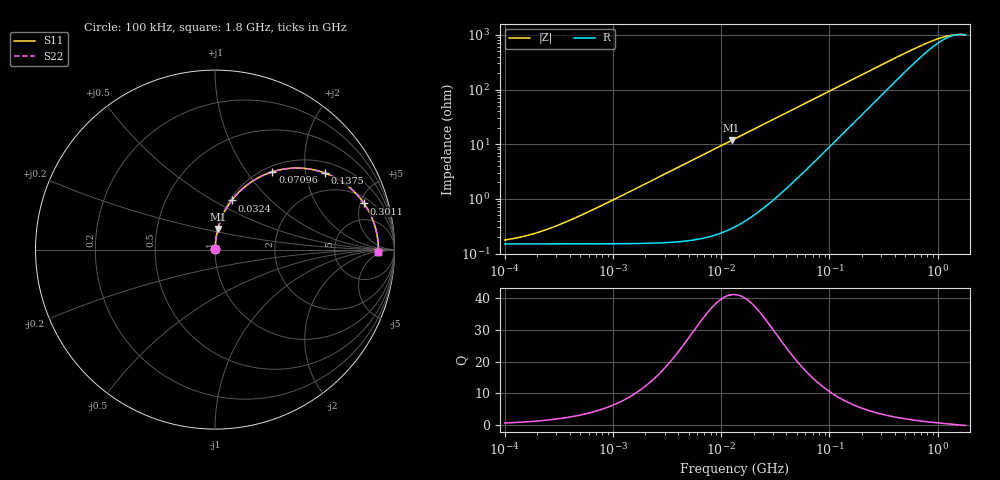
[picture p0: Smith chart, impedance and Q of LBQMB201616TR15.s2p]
! LBQMB201616TR15  S-PARAMETER MODEL  ( General Type )
! Model Generated by TAIYO YUDEN Corporation (http://www.ty-top.com)
! Version 1.0
! TAIYO YUDEN Control No. 191025NI43SB-FBB
! Copyright(c) 2019 TAIYO YUDEN CO.,LTD. All Rights Reserved.
! Product Description (link to TY-COMPAS)
! https://ds.yuden.co.jp/TYCOMPAS/or/detail?pn=LBQMB201616TR15J&u=M
! Products Name : Inductors
! Characteristics :
!  Inductance : 0.15 uH , SRF(min) : 550 MHz , DC Resistance(max) : 0.195 Ohm , Rated Current : 570 mA
!  Case Size : 2.0 x 1.6 / 0.079 x 0.063 [mm/inch] , Thickness : 1.6 / 0.063 [mm/inch]
!  (Conditions: Temperature = 25 degC , DC Bias Current/Voltage = 0A / 0V)
! External Node Assignments :
!  1  o---GGG---o  2
! GND o---------o GND
! Frequency Range : 0.1MHz  -  1800MHz  [ 402 STEP ]
# MHz S RI R 50
! Freq[MHz].  S11 Real  S11 Imag  S21 Real  S21 Imag  S12 Real  S12 Imag  S22 Real  S22 Imag
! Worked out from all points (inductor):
!   401 points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, 100 kHz to 1.8 GHz, reference 50 ohm
!   read as one part in series: L = 150 nH near 479.6 kHz
!   highest Q = 41.1 at 12.47 MHz (marker M1), where L = 150 nH
!   self-resonance near 1.622 GHz
!   S11 on the Smith chart (normalised r, x): 100 kHz: 1.00, +0.00; 32.4 MHz: 1.02, +0.61; 70.96 MHz: 1.09, +1.33; 137.5 MHz: 1.33, +2.57; 301.1 MHz: 2.57, +5.42; 1.8 GHz: 21, -3
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0.1  0.0015 0.00094  0.9985 -0.00094  0.9985 -0.00094  0.0015 0.00094
0.144402  0.0015 0.00136  0.9985 -0.00136  0.9985 -0.00136  0.0015 0.00136
0.21369  0.0015 0.00201  0.9985 -0.00201  0.9985 -0.00201  0.0015 0.00201
0.516129  0.00152 0.00485  0.9985 -0.00485  0.9985 -0.00485  0.00152 0.00485
2.66389  0.00219 0.025  0.9978 -0.025  0.9978 -0.025  0.00219 0.025
6.278453  0.00531 0.0587  0.9947 -0.0587  0.9947 -0.0587  0.00531 0.0587
12.46584  0.0164 0.1152  0.9836 -0.1152  0.9836 -0.1152  0.0164 0.1152
13.41641  0.0187 0.1237  0.9813 -0.1237  0.9813 -0.1237  0.0187 0.1237
21.89777  0.0458 0.1958  0.9542 -0.1958  0.9542 -0.1958  0.0458 0.1958
32.40491  0.0933 0.2738  0.9067 -0.2738  0.9067 -0.2738  0.0933 0.2738
47.95365  0.1811 0.3619  0.8189 -0.3619  0.8189 -0.3619  0.1811 0.3619
69.24595  0.3102 0.4304  0.6898 -0.4304  0.6898 -0.4304  0.3102 0.4304
70.9631  0.3203 0.4337  0.6797 -0.4337  0.6797 -0.4337  0.3203 0.4337
97.57284  0.4616 0.4544  0.5384 -0.4544  0.5384 -0.4544  0.4616 0.4544
137.4876  0.6123 0.4266  0.3877 -0.4266  0.3877 -0.4266  0.6123 0.4266
203.4578  0.7471 0.3488  0.2529 -0.3488  0.2529 -0.3488  0.7471 0.3488
301.0823  0.8305 0.2571  0.1695 -0.2571  0.1695 -0.2571  0.8305 0.2571
357.3983  0.8538 0.2194  0.1462 -0.2194  0.1462 -0.2194  0.8538 0.2194
709.6131  0.8994 0.099  0.1006 -0.099  0.1006 -0.099  0.8994 0.099
1024.694  0.9074 0.0514  0.0926 -0.0514  0.0926 -0.0514  0.9074 0.0514
1374.841  0.9099 0.018  0.0901 -0.018  0.0901 -0.018  0.9099 0.018
1800  0.9102 -0.0113  0.0898 0.0113  0.0898 0.0113  0.9102 -0.0113
